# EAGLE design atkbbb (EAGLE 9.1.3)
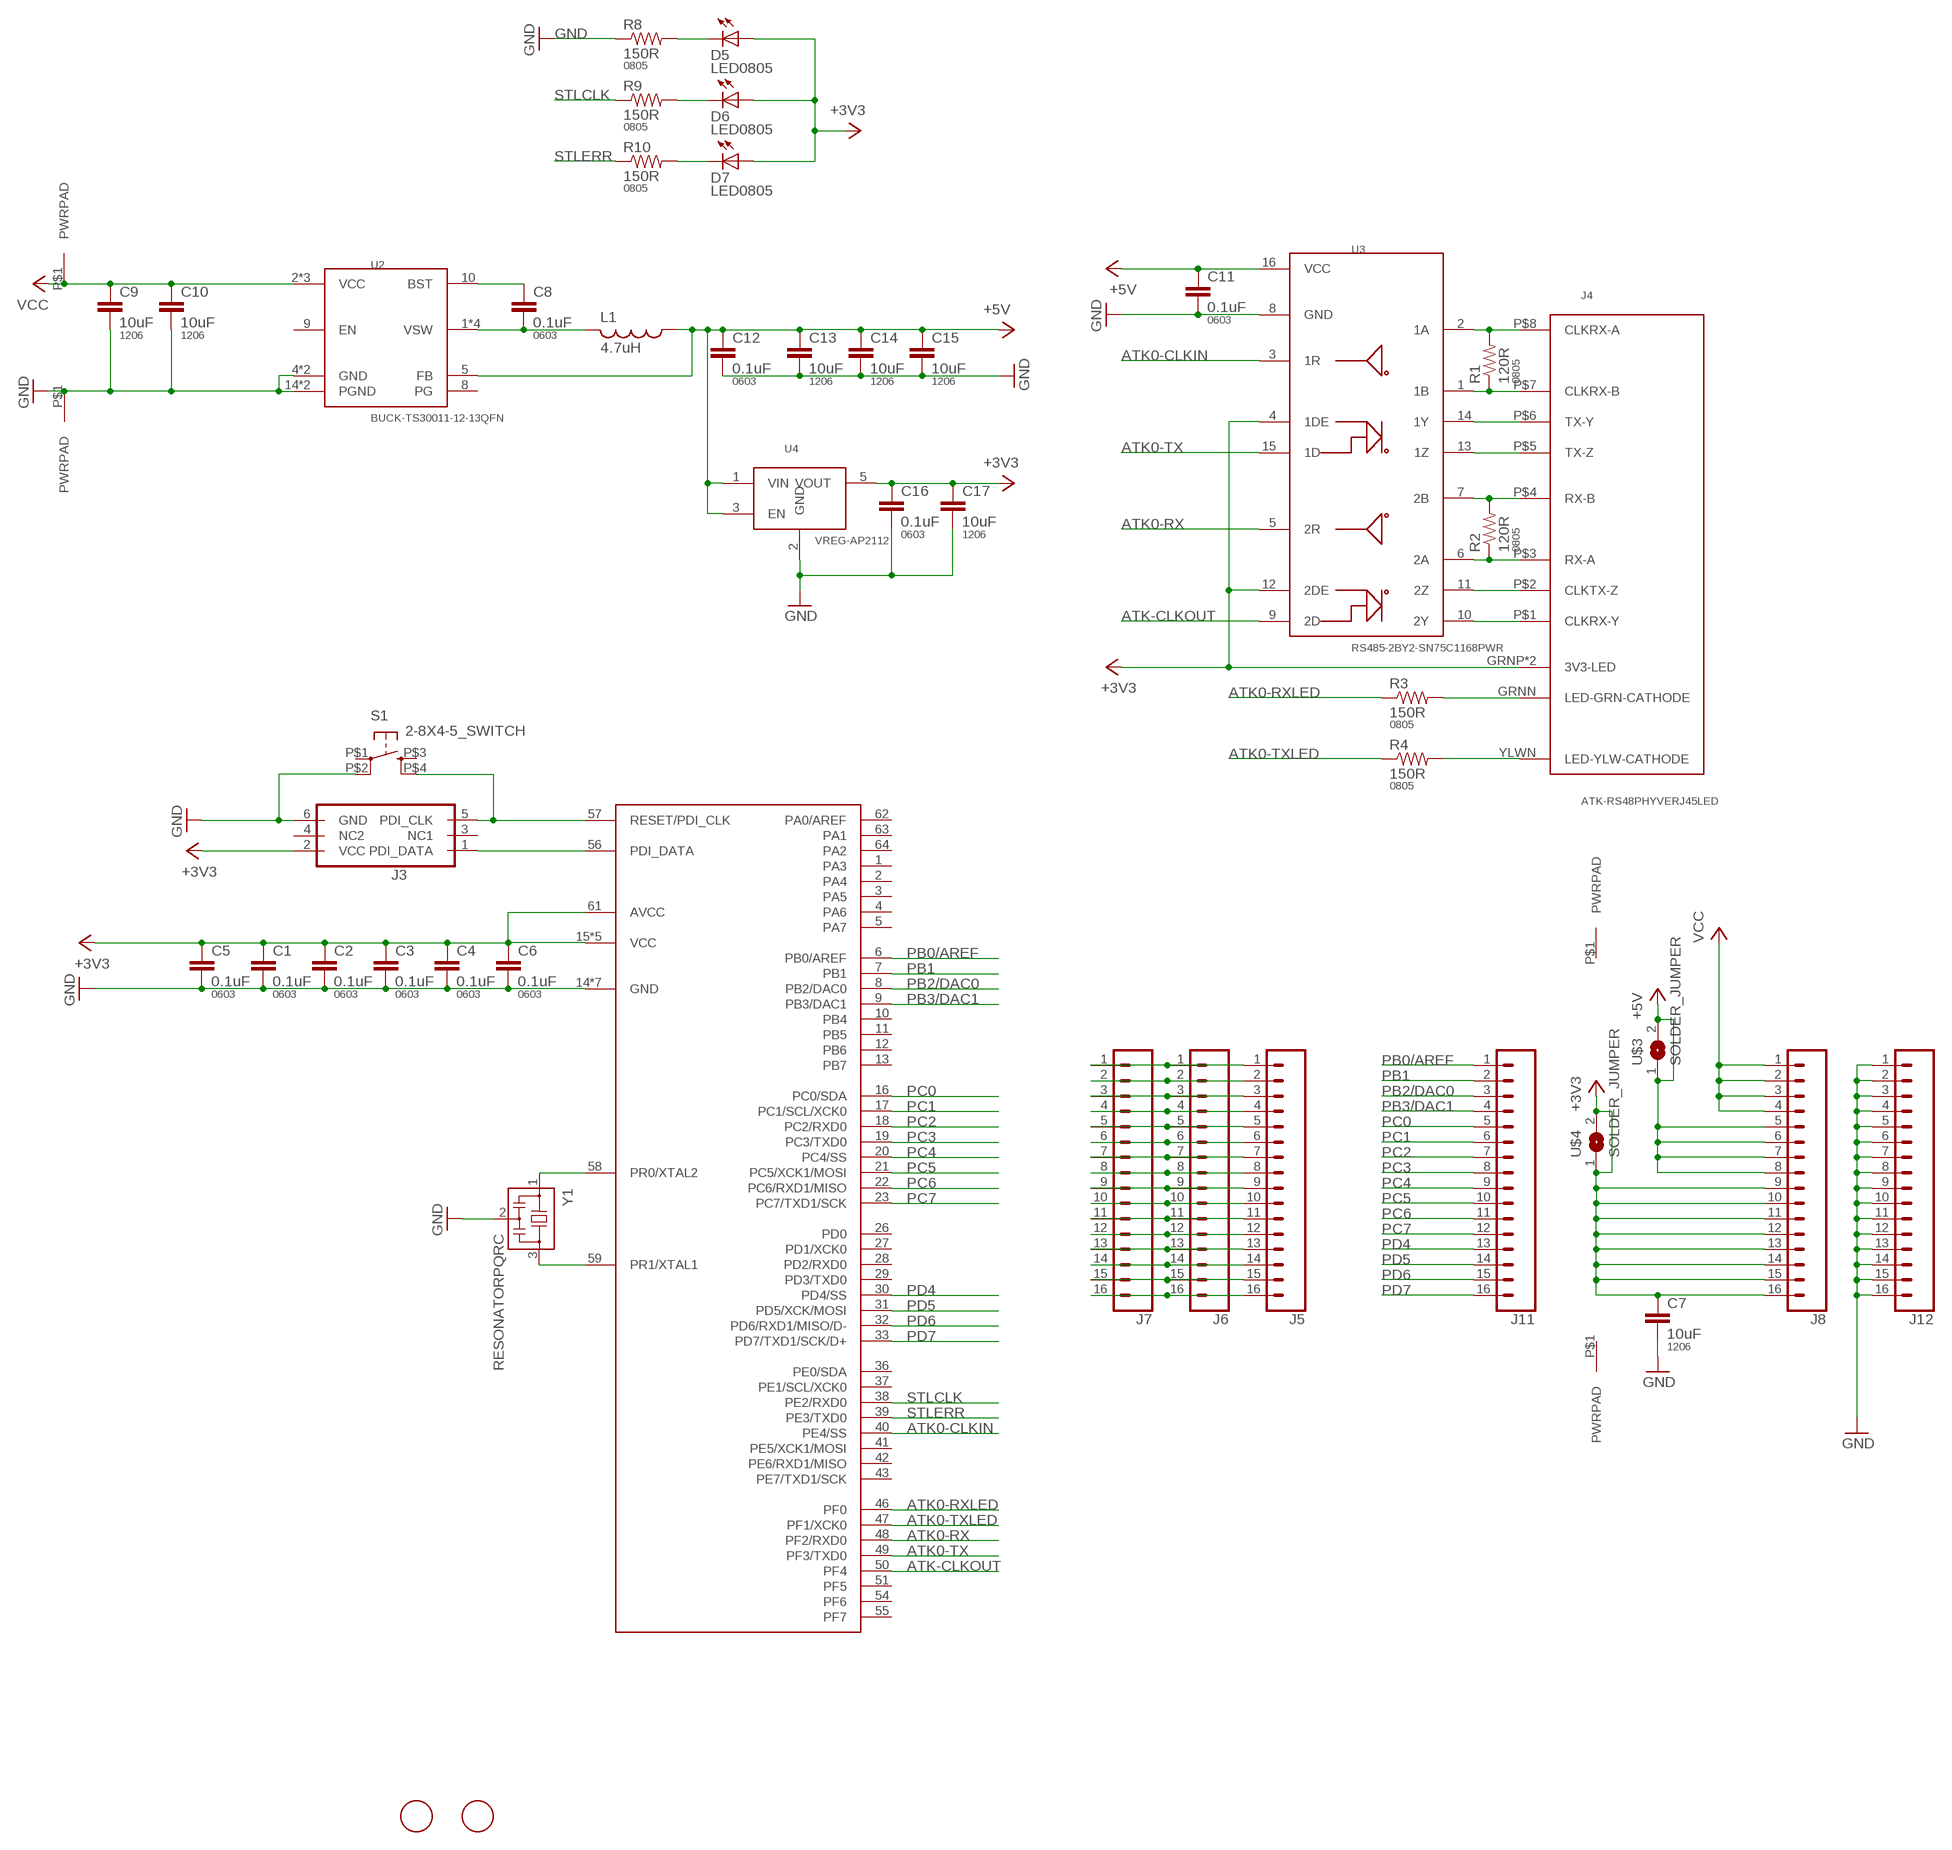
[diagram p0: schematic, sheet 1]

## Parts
C1  0.1uF  CAP0603-CAP  [0603-CAP]
C2  0.1uF  CAP0603-CAP  [0603-CAP]
C3  0.1uF  CAP0603-CAP  [0603-CAP]
C4  0.1uF  CAP0603-CAP  [0603-CAP]
C5  0.1uF  CAP0603-CAP  [0603-CAP]
C6  0.1uF  CAP0603-CAP  [0603-CAP]
C7  10uF  CAP1206  [1206]
C8  0.1uF  CAP0603-CAP  [0603-CAP]
C9  10uF  CAP1206  [1206]
C10  10uF  CAP1206  [1206]
C11  0.1uF  CAP0603-CAP  [0603-CAP]
C12  0.1uF  CAP0603-CAP  [0603-CAP]
C13  10uF  CAP1206  [1206]
C14  10uF  CAP1206  [1206]
C15  10uF  CAP1206  [1206]
C16  0.1uF  CAP0603-CAP  [0603-CAP]
C17  10uF  CAP1206  [1206]
D5  LED0805  [LED0805]
D6  LED0805  [LED0805]
D7  LED0805  [LED0805]
J1  PWRPAD  [PWRPAD_M3-PEM-MOUNT]
J2  PWRPAD  [PWRPAD_M3-PEM-MOUNT]
J3  PDIFEMALE_SMD  [PDI_2X3_SMD]
J4  ATK-RS48PHYVERJ45LED  [RJ45-LED-RJE7318800XXX]
J5  CONN_161X16_NO_SILK  [1X16_NO_SILK]
J6  CONN_161X16_NO_SILK  [1X16_NO_SILK]
J7  CONN_161X16_NO_SILK  [1X16_NO_SILK]
J8  CONN_161X16_NO_SILK  [1X16_NO_SILK]
J9  PWRPADM3  [PWRPAD_3-25MM]
J10  PWRPADM3  [PWRPAD_3-25MM]
J11  CONN_161X16_NO_SILK  [1X16_NO_SILK]
J12  CONN_161X16_NO_SILK  [1X16_NO_SILK]
L1  4.7uH  INDUCTOR  [NRS5020T4R7MMGJ]
R1  120R  RESISTOR0805-RES  [0805]
R2  120R  RESISTOR0805-RES  [0805]
R3  150R  RESISTOR0805-RES  [0805]
R4  150R  RESISTOR0805-RES  [0805]
R8  150R  RESISTOR0805-RES  [0805]
R9  150R  RESISTOR0805-RES  [0805]
R10  150R  RESISTOR0805-RES  [0805]
S1  2-8X4-5_SWITCH  [TACT-SWITCH-KMR6]
U1  ATXMEGA_A3UQFN  [QFN-64-9X9MM]
U2  BUCK-TS30011-12-13QFN  [QFN16-3X3-TI-RTE]
U3  RS485-2BY2-SN75C1168PWR  [TSSOP16]
U4  VREG-AP2112  [SOT23-5]
U$1  FIDUCIAL  [FIDUCIAL_1MM]
U$2  FIDUCIAL  [FIDUCIAL_1MM]
U$3  SOLDER_JUMPER  [SJFAB]
U$4  SOLDER_JUMPER  [SJFAB]
Y1  RESONATORPQRC  [RES_PRQC]

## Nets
+3V3: C1.1 C2.1 C3.1 C4.1 C5.1 C6.1 C7.1 C16.1 C17.1 D5.1(A) D6.1(A) D7.1(A) J3.2(VCC) J4.GRNP(3V3-LED) J4.YLWP(3V3-LED) J8.9 J8.10 J8.11 J8.12 J8.13 J8.14 J8.15 J8.16 U1.15(VCC) U1.25(VCC) U1.35(VCC) U1.45(VCC) U1.53(VCC) U1.61(AVCC) U3.4(1DE) U3.12(2DE) U4.5(VOUT) U$4.1 U$4.2
+5V: C11.1 C12.1 C13.1 C14.1 C15.1 J8.5 J8.6 J8.7 J8.8 L1.1 U2.5(FB) U3.16(VCC) U4.1(VIN) U4.3(EN) U$3.1 U$3.2
ATK0-CLKIN: U1.40(PE4/SS) U3.3(1R)
ATK0-RX: U1.48(PF2/RXD0) U3.5(2R)
ATK0-RXLED: R3.1 U1.46(PF0)
ATK0-TX: U1.49(PF3/TXD0) U3.15(1D)
ATK0-TXLED: R4.1 U1.47(PF1/XCK0)
ATK-CLKOUT: U1.50(PF4) U3.9(2D)
GND: C1.2 C2.2 C3.2 C4.2 C5.2 C6.2 C7.2 C9.2 C10.2 C11.2 C12.2 C13.2 C14.2 C15.2 C16.2 C17.2 J2.P$1(PWRPAD) J3.6(GND) J12.1 J12.2 J12.3 J12.4 J12.5 J12.6 J12.7 J12.8 J12.9 J12.10 J12.11 J12.12 J12.13 J12.14 J12.15 J12.16 R8.1 S1.P$2(P1) U1.14(GND) U1.24(GND) U1.34(GND) U1.44(GND) U1.52(GND) U1.60(GND) U1.P$1(GND) U2.4(GND) U2.14(PGND) U2.15(PGND) U2.TH(GND) U3.8(GND) U4.2(GND) Y1.2
N$1: U1.58(PR0/XTAL2) Y1.1
N$2: U1.59(PR1/XTAL1) Y1.3
N$3: J3.5(PDI_CLK) S1.P$4(S1) U1.57(RESET/PDI_CLK)
N$4: J3.1(PDI_DATA) U1.56(PDI_DATA)
N$5: C8.1 U2.10(BST)
N$6: C8.2 L1.2 U2.1(VSW) U2.12(VSW) U2.13(VSW) U2.16(VSW)
N$7: J4.GRNN(LED-GRN-CATHODE) R3.2
N$8: J4.P$8(CLKRX-A) R1.2 U3.2(1A)
N$9: D5.2(C) R8.2
N$10: D6.2(C) R9.2
N$11: D7.2(C) R10.2
N$12: J4.P$7(CLKRX-B) R1.1 U3.1(1B)
N$13: J4.P$6(TX-Y) U3.14(1Y)
N$14: J4.P$5(TX-Z) U3.13(1Z)
N$15: J4.P$4(RX-B) R2.2 U3.7(2B)
N$16: J4.P$3(RX-A) R2.1 U3.6(2A)
N$17: J4.P$2(CLKTX-Z) U3.11(2Z)
N$18: J4.P$1(CLKRX-Y) U3.10(2Y)
N$19: J4.YLWN(LED-YLW-CATHODE) R4.2
N$20: J5.1 J6.1 J7.1
N$21: J5.2 J6.2 J7.2
N$22: J5.3 J6.3 J7.3
N$23: J5.4 J6.4 J7.4
N$24: J5.5 J6.5 J7.5
N$25: J5.6 J6.6 J7.6
N$26: J5.7 J6.7 J7.7
N$27: J5.8 J6.8 J7.8
N$28: J5.9 J6.9 J7.9
N$29: J5.10 J6.10 J7.10
N$30: J5.11 J6.11 J7.11
N$31: J5.12 J6.12 J7.12
N$32: J5.13 J6.13 J7.13
N$33: J5.14 J6.14 J7.14
N$34: J5.15 J6.15 J7.15
N$35: J5.16 J6.16 J7.16
PB0/AREF: J11.1 U1.6(PB0/AREF)
PB1: J11.2 U1.7(PB1)
PB2/DAC0: J11.3 U1.8(PB2/DAC0)
PB3/DAC1: J11.4 U1.9(PB3/DAC1)
PC0: J11.5 U1.16(PC0/SDA)
PC1: J11.6 U1.17(PC1/SCL/XCK0)
PC2: J11.7 U1.18(PC2/RXD0)
PC3: J11.8 U1.19(PC3/TXD0)
PC4: J11.9 U1.20(PC4/SS)
PC5: J11.10 U1.21(PC5/XCK1/MOSI)
PC6: J11.11 U1.22(PC6/RXD1/MISO)
PC7: J11.12 U1.23(PC7/TXD1/SCK)
PD4: J11.13 U1.30(PD4/SS)
PD5: J11.14 U1.31(PD5/XCK/MOSI)
PD6: J11.15 U1.32(PD6/RXD1/MISO/D-)
PD7: J11.16 U1.33(PD7/TXD1/SCK/D+)
STLCLK: R9.1 U1.38(PE2/RXD0)
STLERR: R10.1 U1.39(PE3/TXD0)
VCC: C9.1 C10.1 J1.P$1(PWRPAD) J8.1 J8.2 J8.3 J8.4 U2.2(VCC) U2.3(VCC) U2.11(VCC)
Unconnected: J3.3(NC1) J3.4(NC2) J9.P$1(PWRPAD) J10.P$1(PWRPAD) S1.P$1(P) S1.P$3(S) U1.1(PA3) U1.2(PA4) U1.3(PA5) U1.4(PA6) U1.5(PA7) U1.10(PB4) U1.11(PB5) U1.12(PB6) U1.13(PB7) U1.26(PD0) U1.27(PD1/XCK0) U1.28(PD2/RXD0) U1.29(PD3/TXD0) U1.36(PE0/SDA) U1.37(PE1/SCL/XCK0) U1.41(PE5/XCK1/MOSI) U1.42(PE6/RXD1/MISO) U1.43(PE7/TXD1/SCK) U1.51(PF5) U1.54(PF6) U1.55(PF7) U1.62(PA0/AREF) U1.63(PA1) U1.64(PA2) U2.8(PG) U2.9(EN)

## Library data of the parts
C1-C6 C8 C11 C12 C16 = borkedlabs-passives:CAP: Capacitor; PACKAGE: 0603
C7 C9 C10 C13-C15 C17 = borkedlabs-passives:CAP: Capacitor; PACKAGE: 1206
D5-D7 = lights:LED: LED
J1 J2 J9 J10 = power:PWRPAD
J3 = microcontrollers:PDI: Multi connection point. Often used as Generic Header-pin footprint for 0.1 inch spaced/style header connections You can populate with any combo of single row headers, but if you'd like an exact match, check these: Header - 2x3 (Male, 0.1") (PRT-12807) Header - 2x3 (Female, 0.1") (PRT-13010) 2x3 Pin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; PROD_ID: CONN-11290
J4 = connector:ATK-RS48PHYVE
J5-J8 J11 J12 = SparkFun-Connectors:CONN_16: Multi connection point. Often used as Generic Header-pin footprint for 0.1 inch spaced/style header connections On any of the 0.1 inch spaced packages, you can populate with these: Break Away Headers - Straight (PRT-00116) Break Away Male Headers - Right Angle (PRT-00553) Female Headers (PRT-00115)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
L1 = power:INDUCTOR
R1-R4 R8-R10 = borkedlabs-passives:RESISTOR: Resistor; PACKAGE: 0805
S1 = passives:2-8X4-5_SWITCH
U1 = microcontrollers:ATXMEGA_A3U
U2 = power:BUCK-TS30011-12-13
U3 = comm:RS485-2BY2-SN75C1168PWR
U4 = power:VREG-AP2112
U$1 U$2 = connector:FIDUCIAL: For use by pick and place machines to calibrate the vision/machine, 1mm
U$3 U$4 = connector:SOLDER_JUMPER
Y1 = passives:RESONATOR

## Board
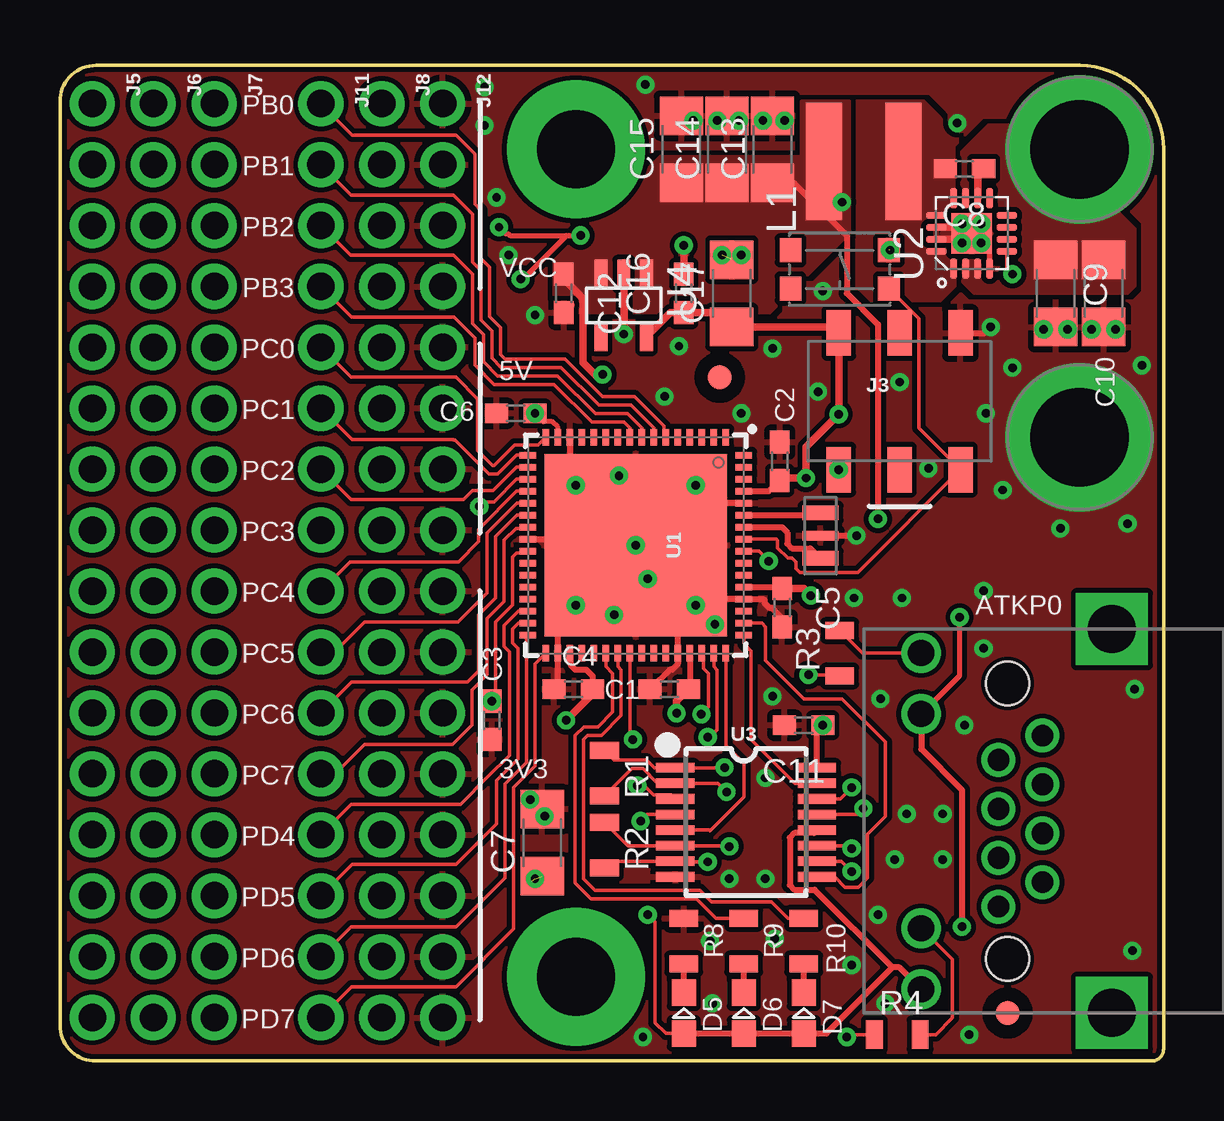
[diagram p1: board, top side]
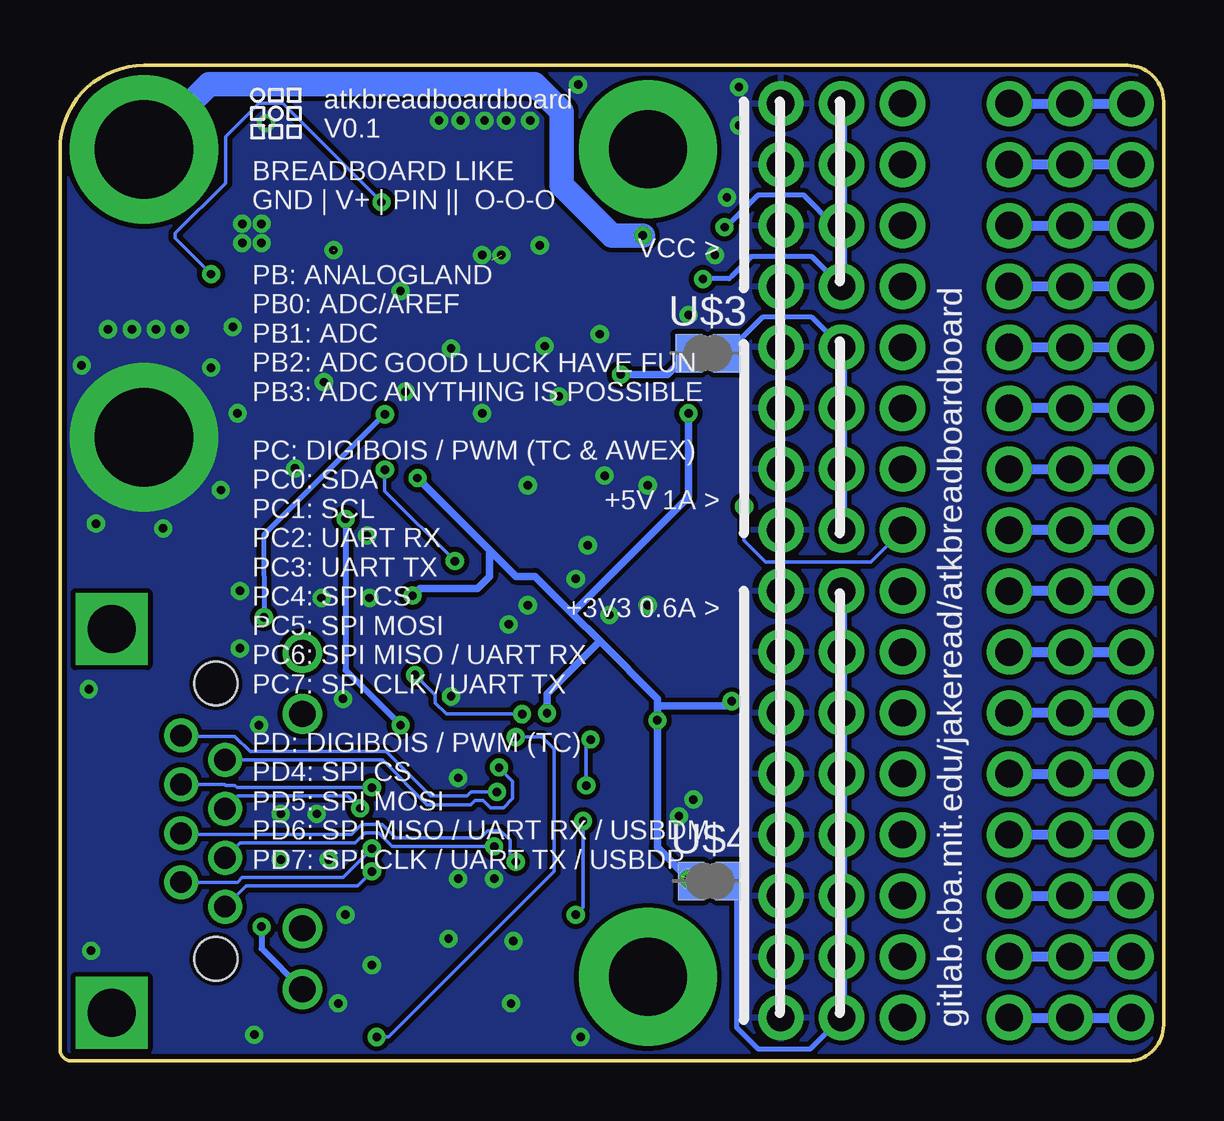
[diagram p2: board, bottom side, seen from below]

Size 46 x 41.5 mm. Coordinates in mm from the lower left corner, seen from the top.
Outline: 42.5,41.5 1.5,41.5 arc90 0,40 0,1.5 arc90 1.5,0 45.5,0 arc90 46,0.5 46,38 arc90 42.5,41.5
Copper layers (1*16): Top 0.035mm / dielectric 1.5mm / Bottom 0.035mm
Design rules "default *": minimum track width 6mil, minimum drill 0.35mm, track to track 8mil, track to pad 8mil, pad to pad 8mil, via to via 8mil, smd to smd 8mil, copper to edge 8mil, drill to drill 8mil, minimum pad ring 10mil, minimum via ring 8mil, stop-mask expansion 4mil, vias tented up to drill 25mil, thermal gap 10mil

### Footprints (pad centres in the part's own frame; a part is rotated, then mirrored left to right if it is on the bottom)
0603-CAP = smd 0.96 x 0.8: 1 -0.8,0; 2 0.8,0
1206 = smd 1.6 x 1.8: 1 -1.4,0; 2 1.4,0
LED0805 = smd 1.1 x 1: 1 -0.85,0; 2 0.85,0
PWRPAD_M3-PEM-MOUNT = drill 4.1 pad 6.2: P$1 0,0
PDI_2X3_SMD = smd 1.02 x 1.9: 1 -2.54,-2.85; 2 -2.54,2.85; 3 0,-2.85; 4 0,2.85; 5 2.54,-2.85; 6 2.54,2.85
RJ45-LED-RJE7318800XXX = drill 1.1: GRNN 7.01,3.6; GRNP 4.47,3.6; YLWN -4.47,3.6; YLWP -7.01,3.6 | drill 0.9: P$1 -3.57,0.38; P$2 -2.55,-1.45; P$3 -1.53,0.38; P$4 -0.51,-1.45; P$5 0.51,0.38; P$6 1.53,-1.45; P$7 2.55,0.38; P$8 3.57,-1.45 | drill 2 square: SHDL1 -8,-4.35; SHDL2 8,-4.35 | hole 1.8: -5.74,0; 5.74,0
1X16_NO_SILK = drill 1.143 pad 1.88: 1 0,0; 2 2.54,0; 3 5.08,0; 4 7.62,0; 5 10.16,0; 6 12.7,0; 7 15.24,0; 8 17.78,0; 9 20.32,0; 10 22.86,0; 11 25.4,0; 12 27.94,0; 13 30.48,0; 14 33.02,0; 15 35.56,0; 16 38.1,0
PWRPAD_3-25MM = drill 3.25 pad 5.75: P$1 0,0
NRS5020T4R7MMGJ = smd 4.9 x 1.5: 1 0,1.65; 2 0,-1.65
0805 = smd 0.7 x 1.2: 1 -0.95,0; 2 0.95,0
TACT-SWITCH-KMR6 = smd 0.9 x 1: P$1 -2.05,0.8; P$2 2.05,0.8; P$3 -2.05,-0.8; P$4 2.05,-0.8
QFN-64-9X9MM = smd 0.7 x 0.275: 1 -4.5,3.75; 2 -4.5,3.25; 3 -4.5,2.75; 4 -4.5,2.25; 5 -4.5,1.75; 6 -4.5,1.25; 7 -4.5,0.75; 8 -4.5,0.25; 9 -4.5,-0.25; 10 -4.5,-0.75; 11 -4.5,-1.25; 12 -4.5,-1.75; 13 -4.5,-2.25; 14 -4.5,-2.75; 15 -4.5,-3.25; 16 -4.5,-3.75; 33 4.5,-3.75; 34 4.5,-3.25; 35 4.5,-2.75; 36 4.5,-2.25; 37 4.5,-1.75; 38 4.5,-1.25; 39 4.5,-0.75; 40 4.5,-0.25; 41 4.5,0.25; 42 4.5,0.75; 43 4.5,1.25; 44 4.5,1.75; 45 4.5,2.25; 46 4.5,2.75; 47 4.5,3.25; 48 4.5,3.75 | smd 0.275 x 0.7: 17 -3.75,-4.5; 18 -3.25,-4.5; 19 -2.75,-4.5; 20 -2.25,-4.5; 21 -1.75,-4.5; 22 -1.25,-4.5; 23 -0.75,-4.5; 24 -0.25,-4.5; 25 0.25,-4.5; 26 0.75,-4.5; 27 1.25,-4.5; 28 1.75,-4.5; 29 2.25,-4.5; 30 2.75,-4.5; 31 3.25,-4.5; 32 3.75,-4.5; 49 3.75,4.5; 50 3.25,4.5; 51 2.75,4.5; 52 2.25,4.5; 53 1.75,4.5; 54 1.25,4.5; 55 0.75,4.5; 56 0.25,4.5; 57 -0.25,4.5; 58 -0.75,4.5; 59 -1.25,4.5; 60 -1.75,4.5; 61 -2.25,4.5; 62 -2.75,4.5; 63 -3.25,4.5; 64 -3.75,4.5 | smd 7.6 x 7.6: P$1 0,0
QFN16-3X3-TI-RTE = smd 0.85 x 0.3: 1 -1.475,0.75; 2 -1.475,0.25; 3 -1.475,-0.25; 4 -1.475,-0.75; 9 1.475,-0.75; 10 1.475,-0.25; 11 1.475,0.25; 12 1.475,0.75 | smd 0.3 x 0.85: 5 -0.75,-1.475; 6 -0.25,-1.475; 7 0.25,-1.475; 8 0.75,-1.475; 13 0.75,1.475; 14 0.25,1.475; 15 -0.25,1.475; 16 -0.75,1.475 | smd 1.7 x 1.7: TH 0,0
TSSOP16 = smd 0.4 x 1.6: 1 -2.225,-2.85; 2 -1.575,-2.85; 3 -0.925,-2.85; 4 -0.275,-2.85; 5 0.375,-2.85; 6 1.025,-2.85; 7 1.675,-2.85; 8 2.325,-2.85; 9 2.325,3.05; 10 1.675,3.05; 11 1.025,3.05; 12 0.375,3.05; 13 -0.275,3.05; 14 -0.925,3.05; 15 -1.575,3.05; 16 -2.225,3.05
SOT23-5 = smd 0.533 x 1.194: 1 -0.95,-1.306; 2 0,-1.306; 3 0.95,-1.306; 4 0.95,1.306; 5 -0.95,1.306
FIDUCIAL_1MM = smd 1 x 1: 1 0,0
SJFAB = smd 1.118 x 1.6: 1 -0.787,0; 2 0.787,0
RES_PRQC = smd 0.6 x 1.5: 1 -0.95,0; 3 0.95,0 | smd 0.4 x 1.5: 2 0,0

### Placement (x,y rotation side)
C1  25.4,15.5 180 top
C2  30,25 90 top
C3  18,14.2 270 top
C4  21.4,15.5 180 top
C5  30.1,18.9 270 top
C6  19,27 180 top
C7  20.1,9.1 90 top
C8  37.7,37.2 180 top
C9  41.5,32 270 top
C10  43.5,32 270 top
C11  31,14 180 top
C12  21,32 270 top
C13  29.7,38 90 top
C14  27.8,38 90 top
C15  25.9,38 90 top
C16  26,32 90 top
C17  28,32 90 top
D5  26,2 90 top
D6  28.5,2 90 top
D7  31,2 90 top
J1  42.5,38 0 top
J2  42.5,26 0 top
J3  35,27.5 0 top
J4  39.5,10 90 top
J5  1.35,39.91 270 top
J6  3.89,39.91 270 top
J7  6.43,39.91 270 top
J8  13.41,39.91 270 top
J9  21.5,3.5 0 top
J10  21.5,38 180 top
J11  10.88,39.91 270 top
J12  15.96,39.91 270 top
L1  33.5,37.5 90 top
R1  22.7,12 270 top
R2  22.7,9 270 top
R3  32.5,17 90 top
R4  34.9,1.1 0 top
R8  26,5 270 top
R9  28.5,5 270 top
R10  31,5 270 top
S1  32.5,33 0 top
U1  24,21.5 270 top
U2  38,34.5 90 top
U3  28.5,10 270 top
U4  23.5,31.5 180 top
U$1  27.5,28.5 0 top
U$2  39.5,2 0 top
U$3  19,29.5 0 bottom
U$4  18.9,7.5 0 bottom
U$6  CBA-LOGO  [CBA-SILK-LOGO]  37,39.5 0 bottom
Y1  31.7,21.9 90 top

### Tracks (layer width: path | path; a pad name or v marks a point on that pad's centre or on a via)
+3V3  (via drill 0.35)  (2 unrouted)
  Top 0.152: U3.4 24.48,10.28 v24.2,10 | v24.5,6.1 24.8,5.8 24.8,1.6 25.25,1.15 D5.1 | U3.12 31.52,9.6 | U1.25 19.42,21.17 19.03,21.17 18.87,21 18.87,19.01 18.16,18.3 18.16,15.16 C3.1
  Top 0.203: J4.GRNP 37.5,16.07 v37.5,18.5 | C6.1 20.14,26.66 20.51,26.66 20.75,26.42 U1.15
  Top 0.254: U1.61 29.55,23.75 C2.1 | C4.1 22.2,16.05 21.93,16.32 21.48,16.32 21.28,16.51 21.28,16.97 U1.35 | U1.45 26.25,15.55 C1.1 | U1.53 30.05,19.75 C5.1 | J4.GRNP 35.9,13 37.6,11.3 v37.6,5.6 | J4.YLWP 34.99,3.9 34.7,3.9 | U3.12 31.43,9.51 30.61,9.51 30.42,9.31 30.42,7.34 30.61,7.14 31.45,7.14 34.7,3.9 | D5.1 D6.1 D7.1 31.95,1.15 32.09,1.29 32.51,1.71 34.7,3.9
  Top 0.305: C2.1 30.1,24.3 v31.1,24.3 31.1,25.6 v32.46,26.96 J3.2 32.21,30.6 C17.1 27.4,31.2 C16.1 25.46,31.2 U4.5 | C5.1 31,19.7 v31.3,19.4 | v21.1,14.2 22.2,15.3 C4.1 | v25.7,14.5 25.7,15 C1.1
  Bottom 0.152: v24.2,10 24.2,6.4 v24.5,6.1
  Bottom 0.203: v37.5,18.5 37.5,21.92 v32.46,26.96 | 13.48,8.13 13.41,8.2 | U$4.2 17.8,7.19 17.8,1.4 16.9,0.5 14.72,0.5 J8.16
  Bottom 0.254: v37.6,5.6 37.6,4.69 J4.YLWP
  Bottom 0.305: v31.3,19.4 31,19.7 28.6,19.7 28.1,20.2 28.1,21.3 | v31.1,24.3 28.1,21.3 | 28.1,21.3 27,20.2 26.2,20.2 24.65,18.65 | 24.65,18.65 23.5,17.5 | 23.5,17.5 21.1,15.1 21.1,14.8 | 21.1,14.8 v21.1,14.2 21.1,8.9 v19.8,7.6 | 23.5,17.5 25.7,15.3 v25.7,14.5 | 21.1,14.8 18.2,14.8 C3.1 | C6.1 19.8,23.5 24.65,18.65
  Bottom 0.406: J8.9 J8.10 J8.11 J8.12 J8.13 13.41,8.2 J8.14 J8.15 J8.16
  Bottom 0.813: U$4.1 U$4.2
  other vias: 18,15 19.8,27
+5V  (via drill 0.35)
  Top 0.152: U2.5 39.48,33.02 v39.7,32.8
  Top 0.254: U3.16 31.55,13.75 C11.1 | C13.1 30.6,36.6 32.8,34.4 32.8,32 34.1,30.7 v34.1,22.6
  Top 0.305: C12.1 21,32.58 21.81,31.77 21.81,31.29 21.8,31.28 21.8,29.12 22.36,28.56 22.56,28.56 v22.62,28.62
  Bottom 0.152: v32.6,35.8 36.73,39.92 37.7,39.92 39.1,38.52 39.1,36.6 41.2,34.5 41.2,34.3 v39.7,32.8
  Bottom 0.203: J8.5 14.66,31 16.71,31 U$3.2
  Bottom 0.254: v34.1,22.6 34.1,16.3 C11.1
  Bottom 0.305: v22.62,28.62 20.67,28.62 U$3.1
  Bottom 0.406: J8.5 J8.6 13.41,25.9 J8.7 J8.8
  Bottom 0.813: U$3.1 U$3.2
  other vias: 31.8,14
  pour Top (no thermals): 32.9,40 30.9,40 30.9,37.7 25,37.7 23,35.7 21.6,35.7 20.6,34.7 20.6,31.2 29.6,31.2 32.9,34.5
ATK0-CLKIN  (via drill 0.35)
  Top 0.152: U3.3 25.48,11.1 24.73,11.1 24.34,11.48 v24.07,11.48 | U1.40 23.75,13.53 v23.88,13.4
  Bottom 0.152: v24.07,11.48 24.07,13.22 v23.88,13.4
ATK0-RX
  Top 0.152: U1.48 27.75,13.15 28.5,12.4 28.5,11 27.1,9.6 27.07,9.62 U3.5
ATK0-RXLED  (via drill 0.35)
  Top 0.152: U1.46 26.83,16.92 26.83,16.36 27.04,16.16 27.04,14.76 v26.74,14.46 | v31.2,16.1 32.45,16.1 R3.1
  Bottom 0.152: v31.2,16.1 30.36,15.26 30.36,14.93 29.89,14.46 v26.74,14.46
ATK0-TX
  Top 0.152: U1.49 28.5,17.4 28.8,17.1 28.8,13.4 30.62,11.57 U3.15
ATK0-TXLED  (via drill 0.35)
  Top 0.152: U1.47 27.25,16.45 27.39,16.31 27.39,13.8 27.09,13.5 v27,13.5 | R4.1 32.9,1.1 v32.8,1
  Bottom 0.152: v27,13.5 25.9,13.5 25.4,13 25.4,7.9 32.3,1 v32.8,1
ATK-CLKOUT
  Top 0.152: U3.9 32.3,7.67 32.73,7.24 33.27,7.24 33.66,7.63 33.66,9.46 34.4,10.2 34.4,13.3 32.6,15.1 31,15.1 29.4,16.7 29.4,18.1 29.25,18.25 U1.50
GND  (via drill 0.35)  (2 unrouted)
  Top 0.203: U2.4 38.75,33.75 v38.4,34.1
  Top 0.254: U1.60 27.25,23.25 v26.5,24 | v21.5,19 20.75,18.25 U1.34 20.75,15.65 C4.2 | U1.24 23.75,21.75 U1.P$1 | U1.14 21.25,24.25 v21.5,24 | C1.2 25.42,16.32 25.52,16.32 25.75,16.55 U1.44 25.75,18.25 v26.5,19 26.75,19.25 U1.52 29.32,19.25 29.37,19.2 29.37,19.08 29.56,18.89 29.68,18.89 30.1,18.47 C5.2 | J3.6 38.55,30.35 v38.8,30.6 | Y1.2 v33.2,21.9
  Top 0.305: U2.14 37.75,34.75 U2.TH | U2.15 37.75,34.25 U2.TH | v38.4,34.1 U2.TH | C12.2 21.3,31.5 | C16.2 v26,34 | U4.2 v23.5,30.3
  other vias: 37.6,34.9 37.6,34.1 38.4,34.9 34.6,33.8 27.6,33.6 28.4,33.6 26.4,39.2 27.4,39.2 28.3,39.2 29.3,39.2 30.2,39.2 24,21.5 41,30.5 42,30.5 43,30.5 44,30.5 29.4,11.8 35.3,10.3 36.8,10.3 36.8,8.4 34.8,8.4 29.7,15.2 27.2,2.4 24.3,1 33.1,19.3 35.1,19.3 34.2,15.1 36.2,24.7 35,28.3 37.4,39.1 24.4,40.7 27.9,7.6 29.4,7.6 38.5,17.2 37.7,14 33,4 34.1,6.1 37.9,1.1 19.6,10.9 20.2,10.2 25.2,27.7 29.7,29.7 31.6,27.9 28.4,27 19.8,31.1 18.7,33.6 18.2,36 17.7,40.6 17.7,39 44.7,4.6 44.8,15.5 39.3,23.8 39.7,28.9 38.6,27 44.5,22.4 45.1,29 41.7,22.2 25.8,29.8 31.8,32.1 34.4,2.4 27.1,5 29.8,5.1 23.1,18.6 24.5,20.1 23.3,24.4 27.3,18.2 38.5,19.6
  pour Top (rank 6): -1,52 -1,-2 48,-2 48,53.5 -0.5,53.5 -0.5,52.5
  pour Bottom (rank 6): -1,54 -1,-2.5 48.5,-2.5 48.5,54
N$1
  Top 0.254: U1.58 30.1,22.25 30.32,22.03 30.32,21.56 30.51,21.37 31.28,21.37 Y1.1
N$2
  Top 0.254: U1.59 31.6,22.75 Y1.3
N$3
  Top 0.152: U1.57 29.86,21.75 29.91,21.7 29.91,21.39 30.34,20.96 30.51,20.96 30.67,20.8 30.67,20.53 30.83,20.37 33.26,20.37 J3.5 35.8,26.39 35.8,30.95 S1.P$4
N$4  (via drill 0.35)
  Top 0.152: U1.56 29.13,21.25 v29.54,20.84
  Bottom 0.152: v29.54,20.84 32.46,23.76 J3.1
  other vias: 32.46,24.65
N$5
  Top 0.305: U2.10 38.25,36.95 C8.1
N$6
  pour Top (rank 3, no thermals): 33.2,40 33.2,32.3 33.8,31.7 36.7,31.7 37.4,32.4 37.4,38.6 36,40
N$7
  Top 0.152: J4.GRNN 33.44,17.01 R3.2
N$8  (via drill 0.35)
  Top 0.152: R1.2 23.85,12.2 24.3,12.2 24.57,11.93 24.57,11.91 24.91,11.57 U3.2 27.43,11.57 v27.79,11.21
  Bottom 0.152: v27.79,11.21 28.86,11.21 29.03,11.04 30.54,11.04 32.4,12.9 38.08,12.9 38.71,13.53 40.91,13.53 J4.P$8
N$9
  Top 0.254: D5.2 R8.2
N$10
  Top 0.254: D6.2 R9.2
N$11
  Top 0.254: D7.2 R10.2
N$12  (via drill 0.35)
  Top 0.152: R1.1 23.09,12.56 24.45,12.56 24.78,12.22 U3.1 v27.69,12.22 v27.7,12.23
  Bottom 0.152: v27.7,12.23 27.13,11.66 27.13,10.94 27.51,10.56 28.06,10.56 28.36,10.86 28.71,10.86 28.88,10.69 30.69,10.69 32.55,12.54 J4.P$7
N$13  (via drill 0.35)
  Top 0.152: U3.14 32.52,10.93 v33,11.4
  Bottom 0.152: v33,11.4 38.62,11.4 38.71,11.49 39.09,11.49 39.13,11.53 J4.P$6
N$14  (via drill 0.35)
  Top 0.152: U3.13 33.23,10.28 v33.49,10.53
  Bottom 0.152: J4.P$5 38.59,11.04 34.2,11.04 34,11.04 v33.49,10.53
N$15  (via drill 0.35)
  Top 0.152: v27,8.3 25.68,8.3 U3.7 22.98,8.32 R2.2
  Bottom 0.152: v27,8.3 27.24,8.54 27.24,9.21 27.63,9.6 28.17,9.6 28.47,9.3 32.01,9.3 32.58,9.87 33.42,9.87 33.85,9.45 40.91,9.45 J4.P$4
N$16  (via drill 0.35)
  Top 0.152: v27.9,8.94 27.87,8.97 U3.6 23.68,8.97 R2.1
  Bottom 0.152: v27.9,8.94 32.15,8.94 32.73,9.52 33.27,9.52 33.7,9.09 38.5,9.09 J4.P$3
N$17  (via drill 0.35)
  Top 0.152: U3.11 32.88,8.97 v33,8.86
  Bottom 0.152: v33,8.86 34.2,7.66 38.4,7.66 38.6,7.45 J4.P$2
N$18  (via drill 0.35)
  Top 0.152: U3.10 32.58,8.32 v33,7.9
  Bottom 0.152: v33,7.9 33.6,7.3 38.25,7.3 J4.P$1
N$19
  Top 0.152: J4.YLWN 37.2,4.23 37.2,1.8 36.5,1.1 R4.2
N$20
  Bottom 0.406: J7.1 J6.1 J5.1
N$21
  Bottom 0.406: J5.2 J6.2 J7.2
N$22
  Bottom 0.406: J7.3 J6.3 J5.3
N$23
  Bottom 0.406: J5.4 J6.4 J7.4
N$24
  Bottom 0.406: J7.5 J6.5 J5.5
N$25
  Bottom 0.406: J5.6 J6.6 J7.6
N$26
  Bottom 0.406: J7.7 J6.7 J5.7
N$27
  Bottom 0.406: J5.8 J6.8 J7.8
N$28
  Bottom 0.406: J5.9 J6.9 J7.9
N$29
  Bottom 0.406: J7.10 J6.10 J5.10
N$30
  Bottom 0.406: J5.11 J6.11 J7.11
N$31
  Bottom 0.406: J7.12 J6.12 J5.12
N$32
  Bottom 0.406: J5.13 J6.13 J7.13
N$33
  Bottom 0.406: J7.14 J6.14 J5.14
N$34
  Bottom 0.406: J5.15 J6.15 J7.15
N$35
  Bottom 0.406: J7.16 J6.16 J5.16
PB0/AREF
  Top 0.152: U1.6 25.17,26.08 25.17,26.47 23.95,27.7 23.2,27.7 22.61,27.7 21.04,29.27 18.54,29.27 18.37,29.44 18.37,30.57 17.91,31.03 17.91,33.09 17.56,33.45 17.56,35.46 17.3,35.71 17.3,37.8 16.5,38.6 12.19,38.6 J11.1
PB1
  Top 0.152: J11.2 12.14,36.1 16.41,36.1 17.2,35.31 17.2,33.3 17.56,32.95 17.56,30.88 18.01,30.42 18.01,29.3 18.39,28.91 20.89,28.91 22.46,27.34 23.8,27.34 24.75,26.39 U1.7
PB2/DAC0
  Top 0.152: J11.3 12.11,33.6 16.4,33.6 17.2,32.8 17.2,30.73 17.66,30.28 17.66,29.15 18.25,28.56 20.75,28.56 22.32,26.98 23.65,26.98 24.25,26.39 U1.8
PB3/DAC1
  Top 0.152: J11.4 12.16,31 16.43,31 17.3,30.13 17.3,29 18.1,28.2 20.6,28.2 22.17,26.63 23.5,26.63 23.75,26.38 U1.9
PC0
  Top 0.152: J11.5 12.12,28.5 16.5,28.5 17.4,27.6 17.4,25.45 18.04,24.81 18.09,24.81 18.95,25.67 19.92,25.67 U1.16
PC1
  Top 0.152: J11.6 12.19,25.9 16.4,25.9 16.41,25.89 16.46,25.89 17.89,24.46 18.24,24.46 19.03,25.25 U1.17
PC2
  Top 0.152: J11.7 12.14,23.4 16.83,23.4 17.21,23.78 18.06,23.78 19.04,24.75 U1.18
PC3  (via drill 0.35)
  Top 0.152: v17.48,23.12 17.66,23.3 18.09,23.3 19.04,24.25 U1.19
  Bottom 0.152: J11.8 12.21,20.8 12.9,20.8 12.91,20.81 16.46,20.81 16.47,20.8 16.6,20.8 17.5,21.7 17.48,21.72 v17.48,23.12
PC4
  Top 0.152: J11.9 12.09,20.81 16.61,20.81 17.45,21.65 17.45,22.16 19.04,23.75 U1.20
PC5
  Top 0.152: J11.10 11.45,17.05 12.7,18.3 16.6,18.3 17.8,19.5 17.8,22.01 19.04,23.25 U1.21
PC6
  Top 0.152: J11.11 12.16,15.8 17,15.8 17.45,16.25 17.45,18.59 18.16,19.3 18.16,21.86 19.05,22.75 U1.22
PC7
  Top 0.152: J11.12 11.47,11.97 12.7,13.2 16.37,13.2 17.17,14.01 17.17,15.47 17.8,16.1 17.8,18.45 18.52,19.16 18.52,21.71 19,22.2 19.45,22.2 U1.23
PD4
  Top 0.152: J11.13 12.14,10.7 16.7,10.7 17.83,11.83 17.83,11.84 18.73,12.74 18.73,17.05 18.52,17.27 18.52,18.15 19.11,18.75 U1.30
PD5
  Top 0.152: J11.14 12.19,8.2 16.5,8.2 18.19,9.89 18.19,11.7 19.09,12.6 19.09,17.2 18.87,17.42 18.87,18 19.12,18.25 U1.31
PD6
  Top 0.152: J11.15 12.12,5.6 16.5,5.6 18.54,7.64 18.54,11.55 19.44,12.45 19.44,17.69 U1.32
PD7
  Top 0.152: J11.16 12.16,3.1 16.5,3.1 18.9,5.5 18.9,11.4 19.8,12.3 19.8,16.55 U1.33
STLCLK
  Top 0.152: R9.1 27.34,5.95 26.54,6.76 22.14,6.76 21.46,7.43 21.46,13.56 21.84,13.94 22.43,13.94 23.04,14.55 23.04,16.15 22.75,16.44 U1.38
STLERR
  Top 0.152: R10.1 30.35,5.95 29.66,6.64 27.15,6.64 26.68,7.11 22.29,7.11 21.82,7.58 21.82,13.42 21.98,13.58 22.57,13.58 23.39,14.4 23.39,16.3 23.25,16.44 U1.39
VCC  (via drill 0.35)
  Top 0.203: v19.2,32.6 19.3,32.6 21.11,34.41 21.2,34.41 | 21.2,34.41 v21.7,34.41 | v18.3,34.76 18.58,34.48 18.68,34.48 18.75,34.41 21.2,34.41
  Bottom 0.203: J8.4 14.66,33.53 17.18,33.53 18.01,32.71 18.11,32.61 v19.19,32.61 v19.2,32.6 | J8.3 13.73,34.83 15,36.1 16.9,36.1 18.24,34.76 v18.3,34.76
  Bottom 0.406: J8.1 J8.2 J8.3 J8.4
  Bottom 1.016: v21.7,34.41 22.98,34.41 25.09,36.52 25.09,37.8 25.09,39.59 26.21,40.71 39.79,40.71 J1.P$1
  pour Top (rank 2, no thermals): 37.6,35.5 37.6,37.9 38.7,39 40.5,39 44.8,34.7 44.8,32.3 44.5,32 38.1,32 37.6,32.5

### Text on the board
tPlace: PB0 | PB1 | PB2 | VCC | PB3 | PC0 | 5V | PC1 | PC2 | PC3 | PC4 | ATKP0 | PC5 | PC6 | 3V3 | PC7 | PD4 | PD5 | PD6 | PD7
bPlace: atkbreadboardboard / V0.1 | BREADBOARD LIKE / GND | V+ | PIN || O-O-O | VCC > | GOOD LUCK HAVE FUN / ANYTHING IS POSSIBLE | +5V 1A > | +3V3 0.6A > | PB: ANALOGLAND / PB0: ADC/AREF / PB1: ADC / PB2: ADC / PB3: ADC / / PC: DIGIBOIS / PWM (TC & AWEX) / PC0: SDA / PC1: SCL / PC2: UART RX / PC3: UART TX / PC4: SPI CS / PC5: SPI MOSI / PC6: SPI MISO / UART RX / PC7: SPI CLK / UART TX / / PD: DIGIBOIS / PWM (TC) / PD4: SPI CS / PD5: SPI MOSI / PD6: SPI MISO / UART RX / USBDM / PD7: SPI CLK / UART TX / USBDP | gitlab.cba.mit.edu/jakeread/atkbreadboardboard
